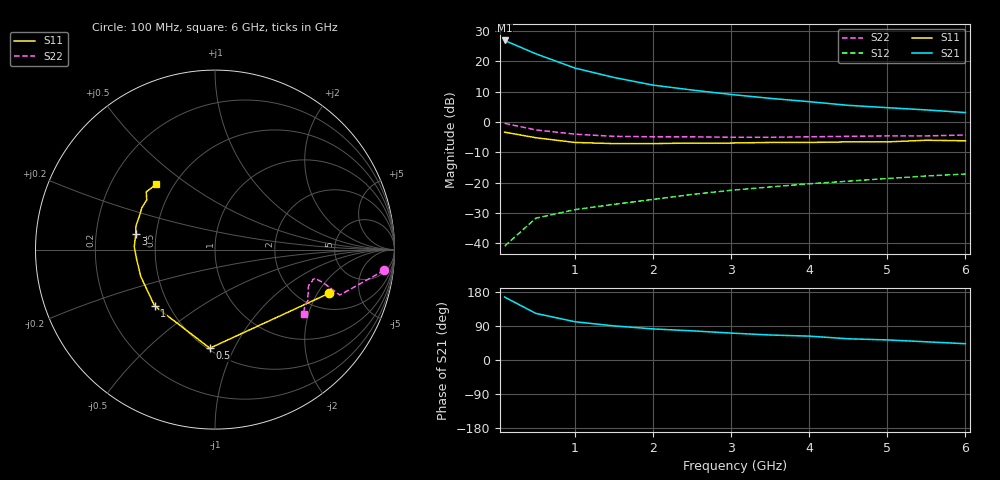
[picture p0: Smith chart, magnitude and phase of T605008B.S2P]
!AT-60500
!S-PARAMETERS at Vce=8V  Ic=10mA.  LAST UPDATED 07-21-92
!OBSOLETED Feb 1994 - nearest replacement: AT-41400
# ghz s ma r 50
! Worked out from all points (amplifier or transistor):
!   13 points, 100 MHz to 6 GHz, reference 50 ohm
!   highest |S21| = 26.9 dB at 100 MHz (marker M1)
!   |S21| within 3 dB of that: start of sweep to 372.8 MHz
!   unconditionally stable (mu >= 1): 1.459 GHz to end of sweep
!   at 1 GHz: K = 0.80, MSG = 23.3 dB, |S12| = -28.9 dB
!   at 3 GHz: K = 1.14, MAG = 13.5 dB, |S12| = -22.5 dB
!   at 6 GHz: K = 1.04, MAG = 8.9 dB, |S12| = -17.1 dB
!   S11 on the Smith chart (normalised r, x): 100 MHz: 2.79, -2.53; 500 MHz: 0.51, -0.81; 1 GHz: 0.42, -0.33; 3 GHz: 0.38, +0.08; 6 GHz: 0.40, +0.38
0.1  0.68 -21.0  22.02 166.0  0.009 80.0  0.95 -7.0
0.5  0.55 -93.0  13.27 123.0  0.026 60.0  0.74 -20.0
1  0.46 -137.0  7.73 101.0  0.036 58.0  0.63 -17.0
1.5  0.44 -160.0  5.41 90.0  0.044 65.0  0.58 -16.0
2  0.44 -173.0  4.05 82.0  0.053 68.0  0.57 -17.0
2.5  0.45 178.0  3.36 77.0  0.064 72.0  0.57 -18.0
3  0.45 169.0  2.84 71.0  0.075 76.0  0.56 -20.0
3.5  0.46 163.0  2.45 66.0  0.085 78.0  0.56 -22.0
4  0.46 157.0  2.16 63.0  0.096 81.0  0.57 -24.0
4.5  0.47 150.0  1.88 56.0  0.106 80.0  0.58 -27.0
5  0.47 144.0  1.72 53.0  0.117 83.0  0.59 -28.0
5.5  0.5 140.0  1.58 48.0  0.129 83.0  0.59 -32.0
6  0.49 132.0  1.43 43.0  0.139 82.0  0.61 -36.0
